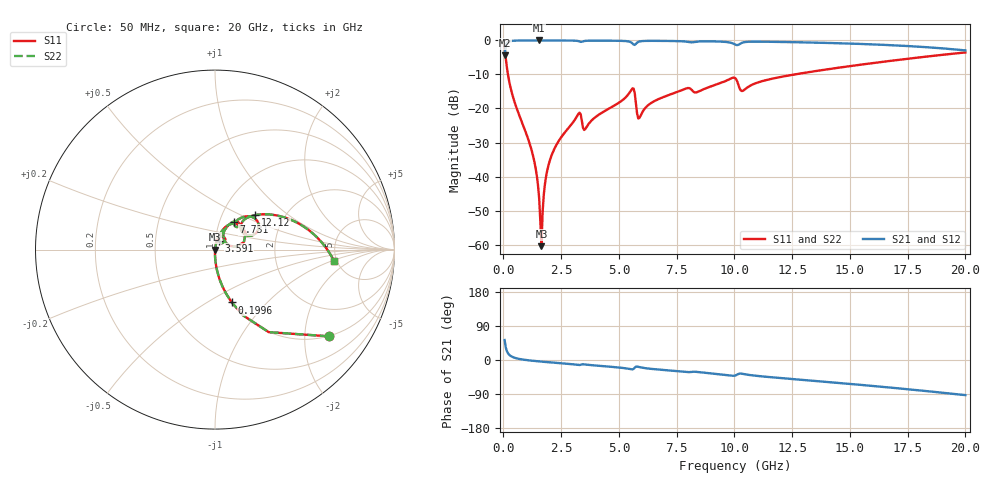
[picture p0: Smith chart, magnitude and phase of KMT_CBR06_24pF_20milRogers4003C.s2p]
! Data measured by Modelithics Inc. support@modelithics.com 813-866-6335
! KEMET CBR0603 24pF, Pad Width= 0.851mm, Pad Length= 0.64mm, Pad Gap= 0.62mm, 20mil Rogers 4003C substrate Data, January 2022
# hz S ma R 50
! 2 Port Network Data from SP1.SP block
! freq  magS11  angS11  magS21  angS21  magS12  angS12  magS22  angS22
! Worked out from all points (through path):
!   401 points, 50 MHz to 20 GHz, reference 50 ohm
!   highest |S21| = -0.01 dB at 1.546 GHz (marker M1); lowest = -4.4 dB at 50 MHz (marker M2)
!   group delay of S21, straight-line fit = 13.2 ps
!   lowest |S11| = -60.5 dB at 1.646 GHz (marker M3), VSWR 1.00, Z = 50.1 + j0.0387 ohm
!   |S11| at or under -10 dB: 195.2 MHz to 12.6 GHz (12.41 GHz wide, 194 % of centre)
!   |S22| runs from -60.5 to -2.0 dB; largest |S21 - S12| = 0
!   S11 on the Smith chart (normalised r, x): 50 MHz: 1.00, -2.62; 199.6 MHz: 1.00, -0.65; 3.591 GHz: 1.04, +0.10; 7.731 GHz: 1.17, +0.37; 12.12 GHz: 1.43, +0.60; 20 GHz: 4.73, -1.09
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5e7  0.7961 -37.3  0.6048 52.6  0.6048 52.6  0.7961 -37.3
1.99625e8  0.3091 -72.4  0.9506 17.5  0.9506 17.5  0.3091 -72.4
4.98875e8  0.1191 -84.2  0.9924 5.5  0.9924 5.5  0.1191 -84.2
1.296875e9  0.01917 -90.1  0.999 -2.3  0.999 -2.3  0.01917 -90.1
1.4465e9  0.01018 -88.8  0.9991 -3.2  0.9991 -3.2  0.01018 -88.8
1.54625e9  0.004753 -84.0  0.9991 -3.7  0.9991 -3.7  0.004753 -84.0
1.646e9  0.0009492 24.0  0.9991 -4.3  0.9991 -4.3  0.0009492 24.0
1.895375e9  0.01226 80.1  0.9989 -5.6  0.9989 -5.6  0.01226 80.1
2.14475e9  0.02305 80.6  0.9986 -6.9  0.9986 -6.9  0.02305 80.6
3.192125e9  0.07769 68.7  0.9852 -12.6  0.9852 -12.6  0.07769 68.7
3.391625e9  0.06696 37.7  0.955 -11.7  0.955 -11.7  0.06696 37.7
3.591125e9  0.05299 66.3  0.988 -12.2  0.988 -12.2  0.05299 66.3
5.53625e9  0.1881 49.6  0.9325 -24.7  0.9325 -24.7  0.1881 49.6
5.885375e9  0.07242 43.8  0.9645 -18.9  0.9645 -18.9  0.07242 43.8
6.73325e9  0.1384 62.7  0.9854 -25.3  0.9854 -25.3  0.1384 62.7
7.73075e9  0.1865 56.4  0.9723 -30.6  0.9723 -30.6  0.1865 56.4
1.0025e10  0.2811 29.9  0.8725 -41.1  0.8725 -41.1  0.2811 29.9
1.037412e10  0.1826 37.3  0.9338 -36.7  0.9338 -36.7  0.1826 37.3
1.211975e10  0.2957 40.6  0.9486 -48.2  0.9486 -48.2  0.2957 40.6
1.336662e10  0.3484 34.4  0.9304 -54.6  0.9304 -54.6  0.3484 34.4
1.670825e10  0.4988 16.0  0.8537 -72.5  0.8537 -72.5  0.4988 16.0
2e10  0.6663 -5.5  0.713 -92.7  0.713 -92.7  0.6663 -5.5
